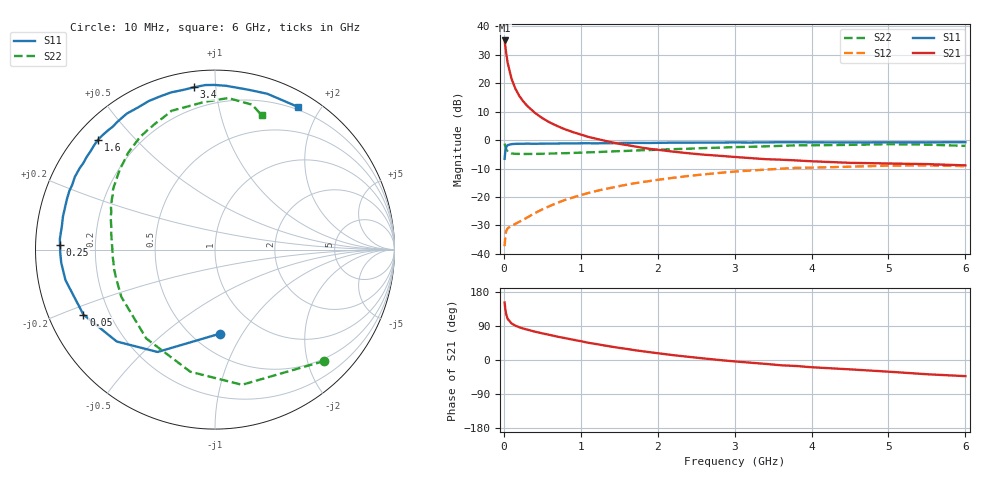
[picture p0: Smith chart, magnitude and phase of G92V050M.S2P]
! SIEMENS Small Signal Semiconductors
! BFG235
! Si NPN RF Bipolar Junction Transistor in SOT223
! VCE = 2 V  IC = 50 mA
! Common Emitter S-Parameters:  July  1994
# GHz  S  MA  R  50
!  f  S11  S21  S12  S22
! GHz  MAG  ANG  MAG  ANG  MAG  ANG  MAG  ANG
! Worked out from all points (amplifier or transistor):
!   40 points, 10 MHz to 6 GHz, reference 50 ohm
!   highest |S21| = 35.0 dB at 10 MHz (marker M1)
!   |S21| within 3 dB of that: start of sweep to 23.76 MHz
!   unconditionally stable (mu >= 1): 491.2 MHz to 1.499 GHz
!   at 200 MHz: K = 0.68, MSG = 22.1 dB, |S12| = -28.7 dB
!   at 1.5 GHz: K = 1.00, MSG = 7.4 dB, |S12| = -16.2 dB
!   at 6 GHz: K = 0.94, MSG = 0.1 dB, |S12| = -9.2 dB
!   S11 on the Smith chart (normalised r, x): 10 MHz: 0.67, -0.81; 50 MHz: 0.11, -0.23; 250 MHz: 0.07, +0.01; 1.6 GHz: 0.06, +0.40; 3.4 GHz: 0.08, +0.88; 6 GHz: 0.17, +1.73
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0.01  0.4685 -86.3  56.38 151.8  0.0137 63.3  0.8696 -45.5
0.02  0.6541 -119.3  43.77 132.8  0.0214 46.8  0.7681 -78.7
0.03  0.7496 -136.9  34.23 120.9  0.0251 37.6  0.6942 -101.4
0.05  0.8177 -153.7  22.69 108.5  0.0283 29.7  0.6261 -127.7
0.1  0.8504 -168.5  11.96 96.6  0.0311 28.2  0.5846 -153.3
0.15  0.8598 -175.1  8.023 90.5  0.0338 32.7  0.5738 -163.7
0.2  0.8622 -178.6  6.006 86.6  0.0368 36.9  0.5725 -169.3
0.25  0.864 178.3  4.838 83.2  0.0397 40.5  0.5701 -173.1
0.3  0.8663 176.0  4.045 80.4  0.0434 44.3  0.5715 -176.2
0.4  0.8632 171.2  3.046 75.0  0.0519 48.5  0.5718 179.6
0.5  0.8669 167.7  2.434 70.3  0.0607 51.3  0.5758 176.4
0.6  0.8679 164.5  2.033 66.1  0.0698 53.4  0.5802 173.5
0.7  0.8717 161.1  1.756 61.5  0.0795 54.0  0.5856 170.9
0.9  0.8735 155.6  1.381 53.5  0.0984 53.6  0.5955 166.4
1.1  0.8801 149.0  1.139 45.4  0.1179 52.2  0.6104 162.0
1.6  0.8943 136.7  0.819 29.2  0.1649 45.4  0.6464 151.8
2.2  0.9032 123.0  0.628 12.8  0.2175 35.3  0.6941 139.7
3.2  0.9071 101.5  0.484 -7.0  0.292 16.0  0.7638 119.7
3.4  0.9118 97.3  0.463 -10.2  0.303 12.0  0.7773 115.3
4.5  0.9099 78.3  0.399 -24.7  0.3414 -8.8  0.8252 94.0
5.5  0.9132 65.4  0.379 -37.6  0.3599 -26.8  0.8335 75.6
6  0.9197 59.7  0.36 -42.6  0.3486 -33.6  0.7919 70.8
